{attribute 'qualified_only'}
{attribute 'strict'}
TYPE E_SboControlState : 
(
	Unselected := 0,
	Select_PerformTest := 1,
	WaitForSelection := 2,
	Ready := 3,
	WaitForActivationTime := 4,
	PerformTest := 5,
	WaitForExecution := 6,
	MirrorBlockedCommand := 7,
	Operate := 8,
	WaitForChange := 9,
	EndSelection := 10
) ;
END_TYPE
